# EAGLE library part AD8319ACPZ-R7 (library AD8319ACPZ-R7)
ANALOG DEVICES - AD8319ACPZ-R7 - Logarithmic Amplifier, 1 Amplifier, 45 dB, 20 ns, LFCSP, 8 Pins Source: Datasheet
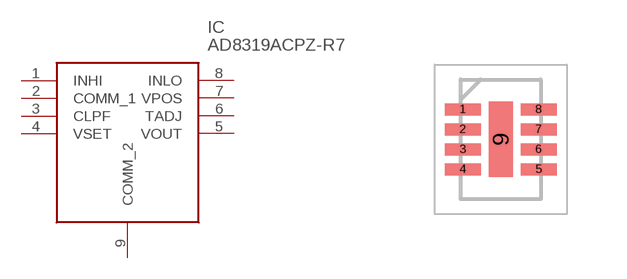
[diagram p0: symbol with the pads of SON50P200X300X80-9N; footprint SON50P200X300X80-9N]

Designator prefix IC

## AD8319ACPZ-R7 (Description: ANALOG DEVICES - AD8319ACPZ-R7 - Logarithmic Amplifier, 1 Amplifier, 45 dB, 20 ns, LFCSP, 8 Pins; Height: 0.8mm; Manufacturer_Name: Analog Devices; Manufacturer_Part_Number: AD8319ACPZ-R7; Mouser_Part_Number: 584-AD8319ACPZ-R7; Mouser_Price-Stock: https://www.mouser.co.uk/ProductDetail/Analog-Devices/AD8319ACPZ-R7?qs=%2FtpEQrCGXCzPBHijRykptA%3D%3D)  [SON50P200X300X80-9N]
1  INHI  in
2  COMM_1  pwr
3  CLPF  out
4  VSET  in
5  VOUT  out
6  TADJ  out
7  VPOS  pwr
8  INLO  in
9  COMM_2  pwr

## Footprint SON50P200X300X80-9N (pad centres in mm)
LFCSP-1
smd 0.9 x 0.3: 1 -0.95,0.75; 2 -0.95,0.25; 3 -0.95,-0.25; 4 -0.95,-0.75; 5 0.95,-0.75; 6 0.95,-0.25; 7 0.95,0.25; 8 0.95,0.75
smd 0.6 x 1.89: 9 0,0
